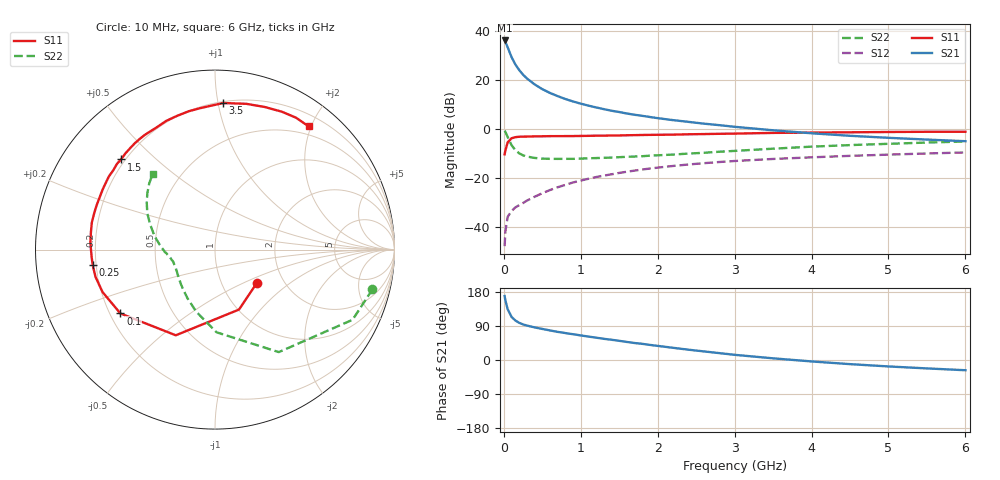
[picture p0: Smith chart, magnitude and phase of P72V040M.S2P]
! SIEMENS Small Signal Semiconductors
! BFP196
! Si NPN RF Bipolar Junction Transistor in SOT143
! VCE = 2 V  IC = 40 mA
! Common Emitter S-Parameters:  May  1996
# GHz  S  MA  R  50
!  f  S11  S21  S12  S22
! GHz  MAG  ANG  MAG  ANG  MAG  ANG  MAG  ANG
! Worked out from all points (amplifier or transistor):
!   36 points, 10 MHz to 6 GHz, reference 50 ohm
!   highest |S21| = 36.0 dB at 10 MHz (marker M1)
!   |S21| within 3 dB of that: start of sweep to 52.3 MHz
!   unconditionally stable (mu >= 1): 458.7 MHz to 4.632 GHz
!   at 250 MHz: K = 0.81, MSG = 26.2 dB, |S12| = -30.3 dB
!   at 1.4 GHz: K = 1.10, MAG = 11.1 dB, |S12| = -18.6 dB
!   at 6 GHz: K = 0.99, MSG = 2.3 dB, |S12| = -9.7 dB
!   S11 on the Smith chart (normalised r, x): 10 MHz: 1.45, -0.60; 100 MHz: 0.24, -0.29; 250 MHz: 0.19, -0.06; 1.5 GHz: 0.18, +0.39; 3.5 GHz: 0.21, +1.04; 6 GHz: 0.37, +1.96
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0.01  0.2985 -39.2  62.95 168.9  0.004 79.3  0.9046 -14.2
0.02  0.3598 -68.2  59.19 157.4  0.008 70.9  0.8606 -27.0
0.05  0.5251 -114.6  45.51 133.9  0.0159 55.4  0.6727 -58.1
0.1  0.6359 -146.0  28.84 113.9  0.0209 47.3  0.4609 -88.9
0.15  0.6697 -159.3  20.35 104.1  0.0247 46.7  0.3622 -106.6
0.2  0.683 -167.2  15.65 98.1  0.0275 48.7  0.313 -119.0
0.25  0.6867 -172.7  12.57 93.9  0.0304 50.8  0.2848 -128.4
0.3  0.6887 -176.7  10.56 90.9  0.034 53.9  0.2699 -134.8
0.4  0.6954 176.8  7.994 86.0  0.0408 57.0  0.2525 -144.4
0.5  0.6982 171.9  6.397 82.0  0.0481 59.1  0.2445 -150.8
0.6  0.7026 167.6  5.344 78.0  0.0559 60.2  0.2417 -155.1
0.7  0.703 163.1  4.599 74.2  0.0637 60.8  0.2414 -158.5
0.9  0.7054 155.9  3.582 68.0  0.0798 60.1  0.242 -163.5
1.1  0.7129 148.9  2.945 61.8  0.095 59.0  0.2483 -166.8
1.5  0.7258 136.2  2.183 50.6  0.1248 54.4  0.2617 -172.2
1.7  0.7372 129.7  1.918 44.8  0.1393 52.0  0.2699 -175.3
2.2  0.7539 116.0  1.49 32.2  0.1732 44.8  0.296 178.2
2.8  0.7844 100.8  1.178 18.2  0.2084 36.3  0.3379 168.7
3.5  0.818 86.8  0.925 4.4  0.2407 26.6  0.3899 158.4
4.5  0.8416 70.7  0.714 -10.9  0.2784 14.7  0.4613 145.5
5.5  0.8625 58.4  0.598 -22.2  0.3114 3.9  0.52 134.8
6  0.8622 52.8  0.554 -27.0  0.3269 -1.9  0.547 129.4
